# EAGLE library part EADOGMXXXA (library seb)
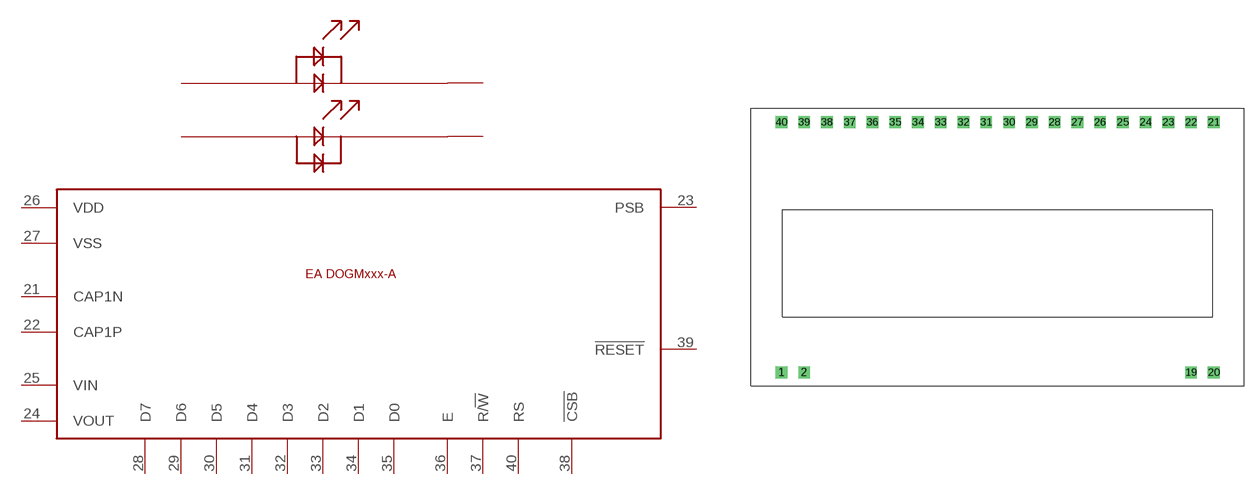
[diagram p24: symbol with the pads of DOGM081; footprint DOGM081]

Designator prefix -

## EADOGMXXXA  [DOGM081]
1  A1
2  C1
19  C2
20  A2
21  CAP1N
22  CAP1P
23  PSB
24  VOUT
25  VIN
26  VDD
27  VSS
28  D7
29  D6
30  D5
31  D4
32  D3
33  D2
34  D1
35  D0
36  E
37  R/!W
38  !CSB
39  !RESET
40  RS

## Footprint DOGM081 (pad centres in mm)
drill 0.8 square: 1 0,0; 2 2.54,0; 19 45.72,0; 20 48.26,0; 21 48.26,27.94; 22 45.72,27.94; 23 43.18,27.94; 24 40.64,27.94; 25 38.1,27.94; 26 35.56,27.94; 27 33.02,27.94; 28 30.48,27.94; 29 27.94,27.94; 30 25.4,27.94; 31 22.86,27.94; 32 20.32,27.94; 33 17.78,27.94; 34 15.24,27.94; 35 12.7,27.94; 36 10.16,27.94; 37 7.62,27.94; 38 5.08,27.94; 39 2.54,27.94; 40 0,27.94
